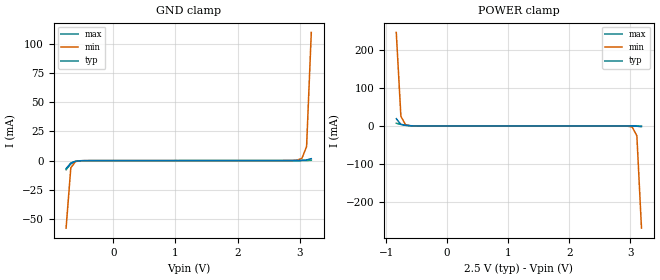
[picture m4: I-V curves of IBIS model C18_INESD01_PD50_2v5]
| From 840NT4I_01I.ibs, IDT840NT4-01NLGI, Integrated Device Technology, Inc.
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| 3.25758e+00   -3.21985e-03   -5.61557e-01   -5.63528e-04
| 3.33333e+00   -1.95987e-02   -1.01660e+00   -1.95169e-03
| 3.40909e+00   -2.66503e-01   -1.47196e+00   -4.76211e-03
| 3.48485e+00   -8.13796e-01   -1.92755e+00   -9.23293e-03
| 3.56061e+00   -1.36142e+00   -2.38330e+00   -3.58634e-02
| 3.63636e+00   -1.90928e+00   -2.83918e+00   -5.06314e-01
| 3.71212e+00   -2.45731e+00   -3.29516e+00   -1.20716e+00
| 3.78788e+00   -3.00546e+00   -3.75121e+00   -1.90820e+00
| 3.86364e+00   -3.55369e+00   -4.20730e+00   -2.60934e+00
| 3.93939e+00   -4.10197e+00   -4.66343e+00   -3.31055e+00
| 4.01515e+00   -4.65027e+00   -5.11958e+00   -4.01177e+00
| 4.09091e+00   -5.19857e+00   -5.57574e+00   -4.71298e+00
| 4.16667e+00   -5.74687e+00   -6.03189e+00   -5.41416e+00
| 4.24242e+00   -6.29514e+00   -6.48804e+00   -6.11528e+00
| 4.31818e+00   -6.84339e+00   -6.94416e+00   -6.81634e+00
| 4.39394e+00   -7.39159e+00   -7.40026e+00   -7.51733e+00
| 4.46970e+00   -7.93974e+00   -7.85633e+00   -8.21823e+00
| 4.54545e+00   -8.48784e+00   -8.31238e+00   -8.91906e+00
| 4.62121e+00   -9.03588e+00   -8.76838e+00   -9.61979e+00
| 4.69697e+00   -9.58387e+00   -9.22435e+00   -1.03204e+01
| 4.77273e+00   -1.01318e+01   -9.68027e+00   -1.10210e+01
| 4.84848e+00   -1.06796e+01   -1.01362e+01   -1.17214e+01
| 4.92424e+00   -1.12274e+01   -1.05920e+01   -1.24218e+01
| 5.00000e+00   -1.17752e+01   -1.10478e+01   -1.31220e+01
[Model] C18_INESD01_PD50_2v5
Model_type   Input
Polarity   Non-Inverting
Vinl = 0.7V
Vinh = 1.7V
|   typ   min   max
C_comp   2pF   1.5pF   2.5pF
|   typ   min   max
[Voltage range]   2.5V   2.375V   2.625V
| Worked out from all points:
|   GND clamp passes 1 mA (typ) near -0.63 V on its own axis
|   POWER clamp passes 1 mA (typ) near -0.63 V on its own axis
[GND_clamp]
|Voltage   I (typ)   I (min)   I (max)
|Note, modeling breaks down at 250mA and above.  This is well beyond the functional   |
|operating range of the device.  Should this scenario occur, catastrophic failure and   |
|possible damage to the device and/or board is of higher concern than the I-V curve   |
|behavior.  The IBIS checker will flag currents in excess of 10A with warnings.  Lines   |
|with currents in excess of 0.35 A have been commented out.  The points still remain|
|available to the user if the user desires to use them.   |
|-2.50000e+00   -2.59051e+01   -2.26503e+01   -3.14096e+01
|-2.42424e+00   -2.47001e+01   -2.16474e+01   -2.98694e+01
|-2.34848e+00   -2.34950e+01   -2.06444e+01   -2.83290e+01
|-2.27273e+00   -2.22897e+01   -1.96413e+01   -2.67883e+01
|-2.19697e+00   -2.10843e+01   -1.86381e+01   -2.52475e+01
|-2.12121e+00   -1.98787e+01   -1.76349e+01   -2.37065e+01
|-2.04545e+00   -1.86730e+01   -1.66315e+01   -2.21652e+01
|-1.96970e+00   -1.74672e+01   -1.56281e+01   -2.06237e+01
|-1.89394e+00   -1.62613e+01   -1.46247e+01   -1.90821e+01
|-1.81818e+00   -1.50552e+01   -1.36212e+01   -1.75402e+01
|-1.74242e+00   -1.38491e+01   -1.26177e+01   -1.59981e+01
|-1.66667e+00   -1.26429e+01   -1.16141e+01   -1.44559e+01
|-1.59091e+00   -1.14366e+01   -1.06106e+01   -1.29135e+01
|-1.51515e+00   -1.02304e+01   -9.60709e+00   -1.13710e+01
|-1.43939e+00   -9.02412e+00   -8.60365e+00   -9.82840e+00
|-1.36364e+00   -7.81792e+00   -7.60030e+00   -8.28573e+00
|-1.28788e+00   -6.61182e+00   -6.59710e+00   -6.74306e+00
|-1.21212e+00   -5.40590e+00   -5.59409e+00   -5.20044e+00
|-1.13636e+00   -4.20024e+00   -4.59132e+00   -3.65800e+00
|-1.06061e+00   -2.99495e+00   -3.58890e+00   -2.11585e+00
|-9.84848e-01   -1.79017e+00   -2.58693e+00   -5.74184e-01
|-9.09091e-01   -5.86135e-01   -1.58556e+00   -3.88946e-02
|-8.33333e-01   -4.29506e-02   -5.85049e-01   -1.60019e-02
-757.6mV  -6.922mA   -57.82mA   -7.788mA
-681.8mV  -2.019mA   -6.114mA   -2.71mA
-606.1mV  -511.5uA   -812.7uA   -604.9uA
-454.5mV  -23.28uA   -29.32uA   -18.42uA
2.803V    56.17uA    63.56uA    59.51uA
2.955V    75.5uA     423.2uA    62.82uA
3.03V     177.1uA    1.883mA    66.35uA
3.106V    606uA      12.06mA    93.9uA
3.182V    1.659mA    109.9mA    302.4uA
| 3.25758e+00   4.02825e-03   8.65269e-01   1.11466e-03
| 3.33333e+00   1.92528e-02   1.92220e+00   2.76019e-03
| 3.40909e+00   2.45489e-01   2.97938e+00   5.14284e-03
| 3.48485e+00   1.44238e+00   4.03678e+00   8.63721e-03
| 3.56061e+00   2.71256e+00   5.09438e+00   3.24306e-02
| 3.63636e+00   3.98300e+00   6.15217e+00   7.13842e-01
| 3.71212e+00   5.25367e+00   7.21013e+00   2.33836e+00
| 3.78788e+00   6.52456e+00   8.26827e+00   3.96319e+00
| 3.86364e+00   7.79565e+00   9.32656e+00   5.58829e+00
| 3.93939e+00   9.06692e+00   1.03850e+01   7.21362e+00
| 4.01515e+00   1.03384e+01   1.14436e+01   8.83917e+00
| 4.09091e+00   1.16100e+01   1.25024e+01   1.04649e+01
| 4.16667e+00   1.28818e+01   1.35613e+01   1.20908e+01
| 4.24242e+00   1.41537e+01   1.46204e+01   1.37169e+01
| 4.31818e+00   1.54258e+01   1.56796e+01   1.53432e+01
| 4.39394e+00   1.66980e+01   1.67391e+01   1.69696e+01
| 4.46970e+00   1.79705e+01   1.77987e+01   1.85962e+01
| 4.54545e+00   1.92431e+01   1.88585e+01   2.02229e+01
| 4.62121e+00   2.05158e+01   1.99185e+01   2.18498e+01
| 4.69697e+00   2.17888e+01   2.09788e+01   2.34769e+01
| 4.77273e+00   2.30620e+01   2.20393e+01   2.51041e+01
| 4.84848e+00   2.43354e+01   2.31002e+01   2.67315e+01
| 4.92424e+00   2.56091e+01   2.41613e+01   2.83591e+01
| 5.00000e+00   2.68830e+01   2.52228e+01   2.99870e+01
[Power_clamp]
|Voltage   I (typ)   I (min)   I (max)
|Note, modeling breaks down at 250mA and above.  This is well beyond the functional   |
|operating range of the device.  Should this scenario occur, catastrophic failure and   |
|possible damage to the device and/or board is of higher concern than the I-V curve   |
|behavior.  The IBIS checker will flag currents in excess of 10A with warnings.  Lines   |
|with currents in excess of 0.35 A have been commented out.  The points still remain|
|available to the user if the user desires to use them.   |
|-2.50000e+00   2.68830e+01   2.34715e+01   3.26734e+01
|-2.42424e+00   2.56091e+01   2.24106e+01   3.10452e+01
|-2.34848e+00   2.43354e+01   2.13500e+01   2.94172e+01
|-2.27273e+00   2.30620e+01   2.02896e+01   2.77894e+01
|-2.19697e+00   2.17888e+01   1.92295e+01   2.61619e+01
|-2.12121e+00   2.05158e+01   1.81696e+01   2.45345e+01
|-2.04545e+00   1.92431e+01   1.71099e+01   2.29074e+01
|-1.96970e+00   1.79705e+01   1.60504e+01   2.12804e+01
|-1.89394e+00   1.66980e+01   1.49911e+01   1.96535e+01
|-1.81818e+00   1.54258e+01   1.39320e+01   1.80269e+01
|-1.74242e+00   1.41537e+01   1.28730e+01   1.64003e+01
|-1.66667e+00   1.28818e+01   1.18142e+01   1.47740e+01
|-1.59091e+00   1.16100e+01   1.07555e+01   1.31478e+01
|-1.51515e+00   1.03384e+01   9.69701e+00   1.15218e+01
|-1.43939e+00   9.06692e+00   8.63865e+00   9.89589e+00
|-1.36364e+00   7.79565e+00   7.58046e+00   8.27021e+00
|-1.28788e+00   6.52456e+00   6.52244e+00   6.64473e+00
|-1.21212e+00   5.25367e+00   5.46458e+00   5.01947e+00
|-1.13636e+00   3.98300e+00   4.40691e+00   3.39447e+00
|-1.06061e+00   2.71256e+00   3.34944e+00   1.76974e+00
|-9.84848e-01   1.44238e+00   2.29219e+00   2.34603e-01
|-9.09091e-01   2.45489e-01   1.23516e+00   1.61447e-02
-833.3mV  19.25mA    247mA      7.144mA
-757.6mV  4.028mA    25.44mA    4.231mA
-681.8mV  1.659mA    3.425mA    2.094mA
-530.3mV  177.1uA    181uA      185.8uA
2.879V    -9.239uA   -76.38uA   -5.392uA
3.03V     -105.5uA   -2.935mA   -10.15uA
3.106V    -511.5uA   -25.77mA   -30.96uA
3.182V    -2.019mA   -269.5mA   -190.7uA
